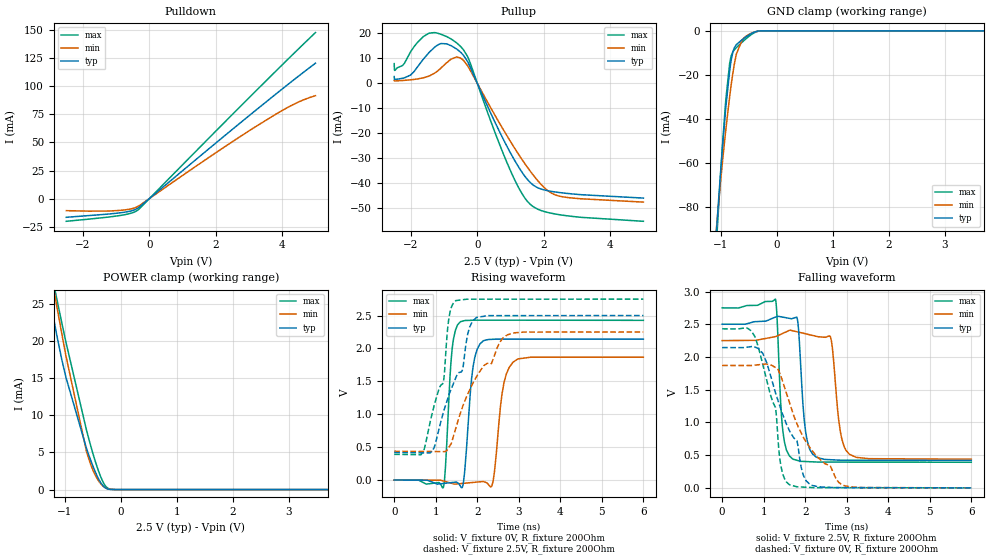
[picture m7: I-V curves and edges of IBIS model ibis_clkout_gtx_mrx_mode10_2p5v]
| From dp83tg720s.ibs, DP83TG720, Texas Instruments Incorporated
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| ibis_clkout_gtx_mrx_mode10_2p5v
[Model]   ibis_clkout_gtx_mrx_mode10_2p5v
Model_type   I/O
Polarity   Non-Inverting
Enable   Active-Low
Vinl = 0.75
Vinh = 1.75
Vmeas = 1.25
Vref = 1.25
Cref = 2pF
Rref = 100000
|   typ   min   max
C_comp   2.97pF   2.94pF   3pF
[Voltage Range]   2.5   2.25   2.75
[Temperature Range]   27   150   -40
[Pullup Reference]   2.5   2.25   2.75
[Pulldown Reference]   0   0   0
[Power Clamp Reference]   2.5   2.25   2.75
[GND Clamp Reference]   0   0   0
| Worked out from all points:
|   slope of the pulldown table from 0 to 0.375 V, typ, clamps not added: 40.2 ohm
|   slope of the pullup table from 0 to 0.375 V, typ, clamps not added: 33.6 ohm
|   GND clamp passes 1 mA (typ) near -0.44 V on its own axis
|   POWER clamp passes 1 mA (typ) near -0.37 V on its own axis
|   falling waveform, V_fixture 2.5V, R_fixture 200Ohm: 20-80 % time 143ps typ, 173ps min, 119ps max; typ from 2.5 V to 0.418 V
|   rising waveform, V_fixture 0V, R_fixture 200Ohm: 20-80 % time 162ps typ, 195ps min, 128ps max; typ from 0 V to 2.14 V
|   rising waveform, V_fixture 2.5V, R_fixture 200Ohm: 20-80 % time 632ps typ, 921ps min, 424ps max; typ from 0.418 V to 2.5 V
|   falling waveform, V_fixture 0V, R_fixture 200Ohm: 20-80 % time 706ps typ, 945ps min, 426ps max; typ from 2.14 V to 0 V
[Pulldown]
|   Voltage   I(typ)   I(min)   I(max)
-2.5V     -16.62mA   -10.71mA   -20.18mA
-925mV    -12.8mA    -10.56mA   -15.22mA
-512.5mV  -10.67mA   -8.868mA   -12.65mA
-347.5mV  -8.464mA   -6.985mA   -10.19mA
1.798V    44.48mA    36.75mA    54mA
3.147V    77.29mA    63.09mA    94.08mA
4.265V    103.8mA    82.73mA    126.8mA
4.633V    112.2mA    87.81mA    137.3mA
5V        120.5mA    91.6mA     147.8mA
[GND Clamp]
|   Voltage   I(typ)   I(min)   I(max)
-2.5V     -675.5mA   -580.7mA   -753.8mA
-1.097V   -98.09mA   -95.14mA   -104.4mA
-1.03V    -73.27mA   -75.43mA   -75.86mA
-962.5mV  -50.24mA   -57.38mA   -49.13mA
-917.5mV  -36.56mA   -46.4mA    -33.41mA
-835mV    -16.75mA   -28.44mA   -13.72mA
-782.5mV  -9.414mA   -18.8mA    -9.429mA
-722.5mV  -6.267mA   -10.55mA   -7.639mA
-617.5mV  -3.988mA   -4.105mA   -5.121mA
-460mV    -1.307mA   -1.167mA   -1.815mA
-265mV    -17.78uA   -43.66uA   -18.24uA
5V        0A         0A         0A
[Pullup]
|   Voltage   I(typ)   I(min)   I(max)
-2.5V     2.676mA    1.082mA    7.872mA
-2.485V   1.505mA    923.3uA    5.155mA
-2.252V   1.977mA    1.098mA    7.082mA
-2.013V   3.235mA    1.359mA    12.48mA
-1.472V   12.01mA    2.778mA    19.94mA
-1.135V   15.74mA    5.587mA    19.86mA
-790mV    15.1mA     9.648mA    17.81mA
-302.5mV  8.958mA    7.249mA    10.98mA
852.5mV   -24.29mA   -20.18mA   -30.56mA
1.587V    -39.78mA   -35.2mA    -48.55mA
2.428V    -43.84mA   -45.21mA   -52.72mA
5V        -46.15mA   -47.75mA   -55.47mA
[POWER Clamp]
|   Voltage   I(typ)   I(min)   I(max)
-2.5V     145mA      109.9mA    192.3mA
-1.42V    32.56mA    36.3mA     36.43mA
-1.248V   24.84mA    28.86mA    29.33mA
-1.15V    20.85mA    24.77mA    25.73mA
-985mV    15.14mA    18.03mA    19.87mA
-617.5mV  5.574mA    5.174mA    8.036mA
-550mV    4.122mA    3.573mA    6.141mA
-460mV    2.4mA      1.958mA    3.831mA
-355mV    861.1uA    726.2uA    1.6mA
-257.5mV  148.6uA    170.2uA    328.1uA
-92.5mV   988.3nA    4.331uA    1.237uA
5V        0A         0A         0A
[Ramp]
R_load = 200
|   typ   min   max
dV/dt_r   1.2848/1.61819e-10   1.12097/1.94579e-10   1.45672/1.2722e-10
dV/dt_f   1.2492/1.42615e-10   1.08767/1.73107e-10   1.41545/1.1893e-10
[Falling Waveform]
V_fixture = 2.5V
V_fixture_min = 2.25V
V_fixture_max = 2.75V
R_fixture = 200Ohm
C_fixture = 0F
|   Time   V(typ)   V(min)   V(max)
0s        2.5V       2.25V      2.75V
1.283ns   2.609V     2.311V     2.884V
1.459ns   2.609V     2.36V      889.2mV
1.703ns   2.59V      2.4V       438.9mV
1.82ns    2.551V     2.383V     417.9mV
2.018ns   827.5mV    2.353V     402.2mV
2.267ns   469.9mV    2.316V     395.1mV
2.614ns   430mV      2.296V     393.8mV
3.069ns   422mV      511.8mV    393.4mV
6ns       418.2mV    437.4mV    391.1mV
[Rising Waveform]
V_fixture = 0V
V_fixture_min = 0V
V_fixture_max = 0V
R_fixture = 200Ohm
C_fixture = 0F
|   Time   V(typ)   V(min)   V(max)
0s        1.798uV    21.54uV    452nV
1.183ns   -52.39mV   -13.81mV   -113.4mV
1.392ns   -37.73mV   -51.34mV   1.969V
1.592ns   -90.44mV   -54.4mV    2.405V
1.898ns   1.717V     -36.4mV    2.429V
2.138ns   2.113V     -22.25mV   2.43V
2.379ns   2.14V      -24.64mV   2.43V
2.596ns   2.143V     1.308V     2.43V
2.857ns   2.142V     1.788V     2.43V
6ns       2.141V     1.868V     2.428V
[Rising Waveform]
V_fixture = 2.5V
V_fixture_min = 2.25V
V_fixture_max = 2.75V
R_fixture = 200Ohm
C_fixture = 0F
|   Time   V(typ)   V(min)   V(max)
0s        418.2mV    437.4mV    391.1mV
715.1ps   413.4mV    434.3mV    453.8mV
962ps     493.9mV    433.2mV    1.132V
1.185ns   1.031V     432.2mV    1.495V
1.317ns   1.292V     498.5mV    2.461V
1.484ns   1.554V     789.1mV    2.728V
1.642ns   1.671V     1.106V     2.741V
1.885ns   2.415V     1.458V     2.749V
2.724ns   2.5V       2.207V     2.749V
6ns       2.5V       2.25V      2.75V
[Falling Waveform]
|Gnd
V_fixture = 0V
V_fixture_min = 0V
V_fixture_max = 0V
R_fixture = 200Ohm
C_fixture = 0F
|   Time   V(typ)   V(min)   V(max)
0s        2.144V     1.87V      2.43V
786.6ps   2.153V     1.875V     2.314V
1.285ns   1.453V     1.84V      1.229V
1.327ns   1.372V     1.825V     926.9mV
1.416ns   1.201V     1.708V     335mV
1.613ns   886.3mV    1.322V     52.26mV
1.802ns   716.9mV    979.7mV    16.66mV
2.025ns   106mV      701.5mV    9.302mV
2.9ns     3.746mV    43.24mV    2.922mV
6ns       1.757uV    21.54uV    541.6nV
